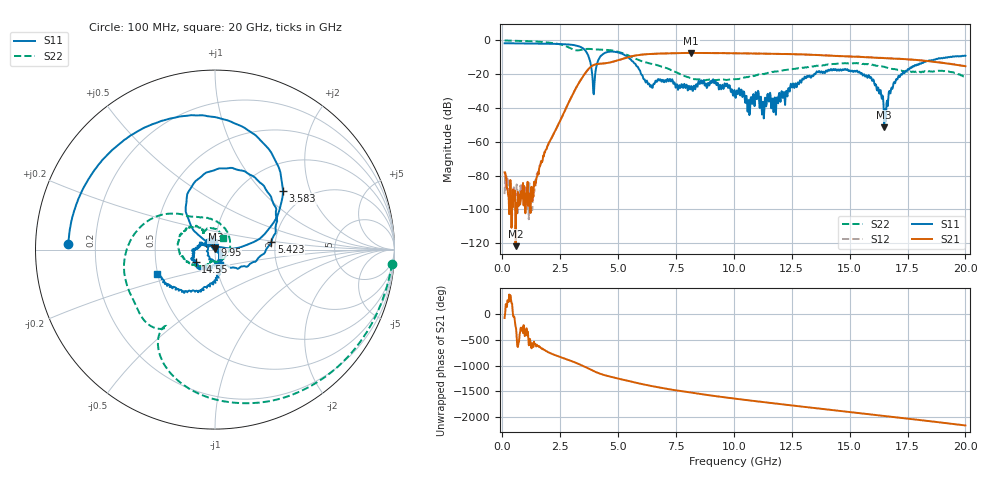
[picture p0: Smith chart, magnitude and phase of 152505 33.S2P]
!  2-Port S-parameters saved by WinCal
! VAR MeasName=S-Parameters (CALIBRATED_DATA) read from VNA (N5230C)
! VAR MeasDate=4/10/2015 9:31:41 AM
! VAR NAME=152505 33
! VAR FILENAME=152505 33.S2P
! VAR DATE=4/10/2015 9:31:41 AM
! VAR PHYS_PORTS=1,2
# Hz S DB R 50
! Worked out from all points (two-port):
!   801 points, 100 MHz to 20 GHz, reference 50 ohm
!   highest |S21| = -7.44 dB at 8.159 GHz (marker M1); lowest = -121.7 dB at 572.6 MHz (marker M2)
!   |S21| within 3 dB of the highest: 5.329 GHz to 16.35 GHz (11.02 GHz wide, 102 % of centre)
!   lowest |S11| = -51.5 dB at 16.49 GHz (marker M3), VSWR 1.01, Z = 50.2 + j0.177 ohm
!   |S11| at or under -10 dB: 3.737 GHz to 4.215 GHz (477.9 MHz wide, 12 % of centre); 5.427 GHz to 19.24 GHz (13.82 GHz wide, 112 % of centre)
!   |S22| runs from -23.7 to -0.1 dB; largest |S21 - S12| = 0.0063
!   S11 on the Smith chart (normalised r, x): 100 MHz: 0.10, +0.02; 3.583 GHz: 1.52, +1.33; 5.423 GHz: 1.91, +0.18; 9.95 GHz: 0.99, +0.05; 14.55 GHz: 0.80, -0.11; 20 GHz: 0.50, -0.15
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1e8  -1.75 177.6  -78.10 -81.9  -90.94 117.5  -0.08 -4.6
5.72625e8  -1.78 166.4  -121.74 112.2  -91.80 92.9  -0.28 -23.4
1.493e9  -1.91 143.5  -80.72 122.5  -78.96 101.9  -0.74 -60.8
2.63725e9  -2.29 106.8  -43.50 -135.9  -43.66 -136.0  -2.94 -112.3
3.43325e9  -4.29 57.7  -22.45 82.8  -22.46 83.1  -5.56 -123.4
3.5825e9  -6.01 40.8  -19.43 52.8  -19.43 52.8  -5.17 -127.9
3.955625e9  -31.92 117.4  -14.55 -29.1  -14.57 -28.9  -5.31 -143.2
4.3785e9  -7.87 103.4  -13.66 -100.6  -13.70 -100.8  -5.55 -159.2
5.42325e9  -9.97 7.6  -10.05 144.8  -10.04 144.9  -8.80 148.5
6.393375e9  -27.51 -159.4  -8.08 48.3  -8.08 48.4  -13.78 117.8
6.741625e9  -22.88 135.0  -7.87 18.9  -7.87 18.7  -14.86 102.6
8.1595e9  -27.01 115.2  -7.44 -84.6  -7.44 -84.6  -22.50 -12.7
9.9505e9  -31.90 97.8  -7.63 166.4  -7.65 166.2  -22.96 -106.4
1.005e10  -32.19 91.7  -7.64 160.7  -7.67 160.7  -22.94 -107.9
1.171662e10  -42.51 40.6  -7.98 71.1  -8.01 70.8  -18.70 -128.8
1.338325e10  -20.83 -90.2  -8.59 -15.7  -8.54 -15.4  -15.43 -155.5
1.455238e10  -18.00 -147.7  -9.31 -74.5  -9.31 -74.3  -13.70 176.0
1.59205e10  -21.77 154.4  -10.14 -142.9  -10.07 -142.8  -14.23 141.1
1.649262e10  -51.50 41.4  -10.50 -171.0  -10.48 -171.1  -15.64 127.4
1.669162e10  -30.79 -42.0  -10.63 178.8  -10.62 178.5  -16.58 124.5
1.77115e10  -15.41 -88.3  -11.48 125.9  -11.40 125.5  -18.64 122.0
2e10  -9.14 -157.1  -15.32 3.4  -15.31 3.1  -22.17 53.6
